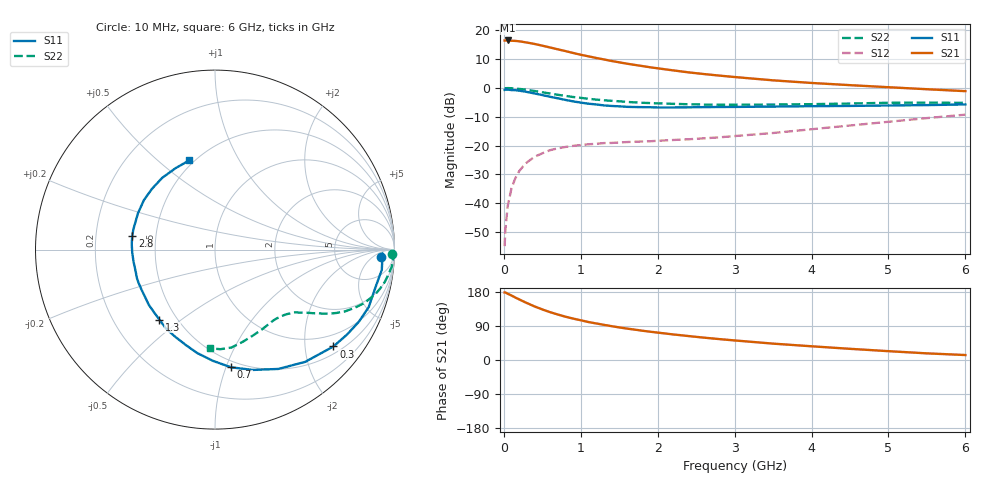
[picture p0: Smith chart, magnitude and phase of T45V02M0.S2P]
! Infineon Technologies  Discrete & RF Semiconductors
! BFR182T
! Si NPN RF Bipolar Junction Transistor in SC75
! VCE = 5 V  IC = 2 mA
! Common Emitter S-Parameters:  October  1999
# GHz  S  MA  R  50
!  f  S11  S21  S12  S22
! GHz  MAG  ANG  MAG  ANG  MAG  ANG  MAG  ANG
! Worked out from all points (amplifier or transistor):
!   36 points, 10 MHz to 6 GHz, reference 50 ohm
!   highest |S21| = 16.5 dB at 50 MHz (marker M1)
!   |S21| within 3 dB of that: start of sweep to 689.4 MHz
!   unconditionally stable (mu >= 1): 2.025 GHz to 4.355 GHz
!   at 250 MHz: K = 0.14, MSG = 21.6 dB, |S12| = -27.2 dB
!   at 1.4 GHz: K = 0.77, MSG = 14.2 dB, |S12| = -19.1 dB
!   at 6 GHz: K = 0.83, MSG = 4.1 dB, |S12| = -9.3 dB
!   lowest NFmin = 1.10 dB at 450 MHz
!   S11 on the Smith chart (normalised r, x): 10 MHz: 20, -10; 300 MHz: 0.67, -2.65; 700 MHz: 0.45, -1.04; 1.3 GHz: 0.40, -0.42; 2.8 GHz: 0.37, +0.07; 6 GHz: 0.47, +0.64
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0.01  0.9229 -2.4  6.64 178.3  0.0018 79.3  0.9888 -1.3
0.02  0.9342 -1.3  6.648 178.3  0.0035 92.1  0.9906 -1.0
0.05  0.9361 -6.9  6.666 174.9  0.0089 88.3  0.9939 -2.8
0.1  0.9185 -13.2  6.592 170.1  0.0183 84.6  0.9895 -5.5
0.15  0.9143 -20.5  6.55 164.8  0.0273 78.2  0.9755 -8.3
0.2  0.8965 -26.7  6.444 159.8  0.0361 75.7  0.9629 -10.8
0.3  0.8523 -39.3  6.133 150.3  0.0511 69.0  0.9275 -15.5
0.4  0.8024 -51.2  5.794 141.3  0.0641 62.8  0.885 -19.6
0.5  0.753 -62.0  5.414 133.5  0.0734 57.9  0.8422 -22.7
0.6  0.703 -72.5  5.037 126.3  0.0832 53.8  0.8009 -25.5
0.7  0.662 -82.2  4.683 120.1  0.0896 50.9  0.7621 -27.6
0.9  0.585 -99.7  4.044 109.3  0.0989 45.7  0.6965 -30.8
1.1  0.5332 -114.8  3.537 100.2  0.1055 42.9  0.6488 -33.1
1.3  0.4981 -128.4  3.129 92.8  0.1105 41.3  0.6116 -35.1
1.6  0.4703 -146.1  2.637 82.9  0.1152 40.7  0.5725 -37.6
1.9  0.463 -160.2  2.285 74.7  0.1189 42.2  0.5467 -40.7
2.2  0.4588 -171.5  2.018 67.5  0.1251 44.3  0.5302 -43.5
2.8  0.4673 170.8  1.639 55.2  0.139 49.5  0.5112 -50.7
3.5  0.4747 154.7  1.355 43.2  0.1654 55.2  0.5159 -59.4
4.5  0.4877 136.2  1.118 29.5  0.223 58.8  0.5367 -73.3
5.5  0.504 115.8  0.95 17.5  0.2999 57.2  0.5557 -86.8
6  0.5174 106.1  0.88 13.1  0.3439 54.3  0.551 -93.0
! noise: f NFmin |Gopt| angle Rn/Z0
0.45  1.1  0.42  29  0.36
0.9  1.2  0.4  58  0.3
1.8  1.85  0.32  126  0.22
